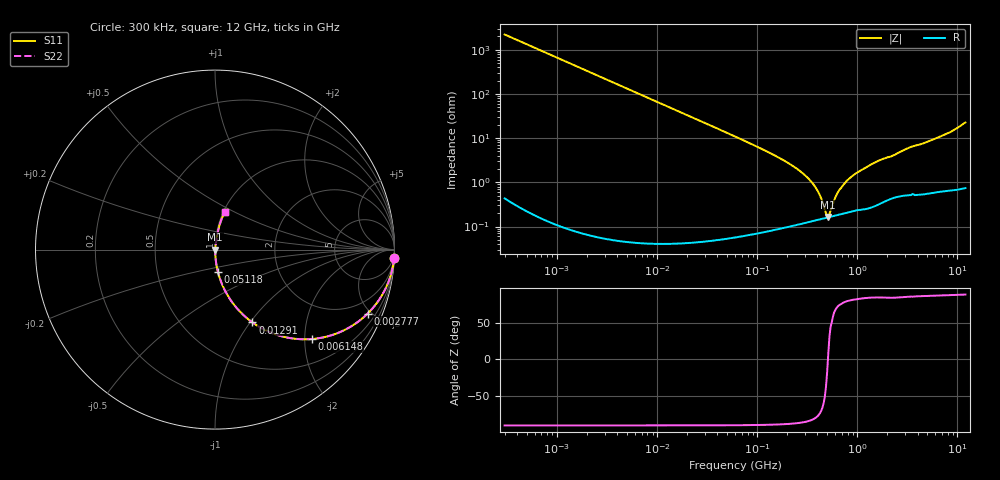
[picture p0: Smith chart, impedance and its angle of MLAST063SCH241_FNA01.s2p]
! MLAST063SCH241_FNA01  S-PARAMETER MODEL  ( General Type )
! Model Generated by TAIYO YUDEN Corporation (http://www.ty-top.com)
! Version 1.0
! TAIYO YUDEN Control No. 160830
! Copyright(c) 2016 TAIYO YUDEN CO.,LTD. All Rights Reserved.
! Product Description (link to TY-COMPAS)
! https://ds.yuden.co.jp/TYCOMPAS/or/detail?pn=MLAST063SCH241JFNA01&u=M
! Products Name : Multilayer Ceramic Capacitors
! Characteristics :
!  Capacitance : 240 pF , Rated Voltage : 25V , TCC : CH / C0H
!  Case Size : 0.6 x 0.3 / 0.024 x 0.012 [mm/inch] , Thickness : 0.3 / 0.012 [mm/inch]
!  (Conditions: Temperature = 25 degC , DC Bias Current/Voltage = 0A / 0V)
! External Node Assignments :
!  1  o---| |---o  2
! GND o---------o GND
! Frequency Range : 0.3MHz  -  12000MHz  [ 401 STEP ]
# MHz S RI R 50
! Freq[MHz].  S11 Real  S11 Imag  S21 Real  S21 Imag  S12 Real  S12 Imag  S22 Real  S22 Imag
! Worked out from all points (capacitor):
!   401 points, 300 kHz to 12 GHz, reference 50 ohm
!   read as one part in series: C = 240 pF near 316.3 kHz
!   lowest |Z| = 163 mohm at 512.9 MHz (marker M1)
!   series resonance near 508.6 MHz, so ESL is about 410 pH
!   S11 on the Smith chart (normalised r, x): 300 kHz: 1, -44; 2.777 MHz: 1.00, -4.78; 6.148 MHz: 1.00, -2.16; 12.91 MHz: 1.00, -1.03; 51.18 MHz: 1.00, -0.26; 12 GHz: 1.01, +0.45
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0.3  0.9979 -0.0451  0.00205 0.0451  0.00205 0.0451  0.9979 -0.0451
0.799488  0.9857 -0.1188  0.0143 0.1188  0.0143 0.1188  0.9857 -0.1188
1.769972  0.9335 -0.2491  0.0665 0.2491  0.0665 0.2491  0.9335 -0.2491
2.776859  0.8508 -0.3562  0.1492 0.3562  0.1492 0.3562  0.8508 -0.3562
6.147639  0.5377 -0.4984  0.4623 0.4984  0.4623 0.4984  0.5377 -0.4984
10.44266  0.2873 -0.4522  0.7127 0.4522  0.7127 0.4522  0.2873 -0.4522
12.90781  0.2088 -0.4061  0.7912 0.4061  0.7912 0.4061  0.2088 -0.4061
23.11883  0.0761 -0.2644  0.9239 0.2644  0.9239 0.2644  0.0761 -0.2644
51.18236  0.0167 -0.126  0.9833 0.126  0.9833 0.126  0.0167 -0.126
60  0.0123 -0.1076  0.9877 0.1076  0.9877 0.1076  0.0123 -0.1076
197.6437  0.00177 -0.0284  0.9982 0.0284  0.9982 0.0284  0.00177 -0.0284
278.9009  0.00143 -0.0166  0.9986 0.0166  0.9986 0.0166  0.00143 -0.0166
353.9943  0.00141 -0.00965  0.9986 0.00965  0.9986 0.00965  0.00141 -0.00965
414.98  0.00146 -0.00535  0.9985 0.00535  0.9985 0.00535  0.00146 -0.00535
486.4723  0.00157 -0.00118  0.9984 0.00118  0.9984 0.00118  0.00157 -0.00118
512.9422  0.00161 0.000236  0.9984 -0.000236  0.9984 -0.000236  0.00161 0.000236
634.0297  0.00185 0.00548  0.9982 -0.00548  0.9982 -0.00548  0.00185 0.00548
826.3444  0.00225 0.0118  0.9978 -0.0118  0.9978 -0.0118  0.00225 0.0118
1403.667  0.00338 0.0258  0.9966 -0.0258  0.9966 -0.0258  0.00338 0.0258
2088.533  0.00543 0.0367  0.9946 -0.0367  0.9946 -0.0367  0.00543 0.0367
8064.993  0.0228 0.1266  0.9772 -0.1266  0.9772 -0.1266  0.0228 0.1266
12000  0.0548 0.2118  0.9452 -0.2118  0.9452 -0.2118  0.0548 0.2118
